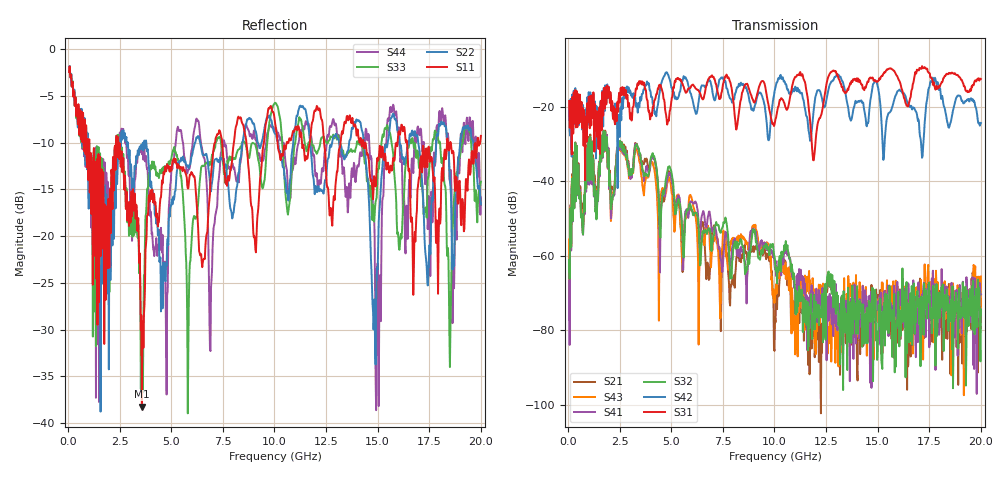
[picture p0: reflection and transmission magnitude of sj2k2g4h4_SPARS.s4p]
! FILE: E:\users\goganessyan\GBX_Backplane\FR408_backplane\1m_OUTBOUND_FEXT\sj2k2g4h4_SPARS.s4p
# MHZ S RI R 50.00
! FREQ  S11  S12  S13  S14
!  S21  S22  S23  S24
!  S31  S32  S33  S34
!  S41  S42  S43  S44
!  REAL  IMAG  REAL  IMAG  REAL  IMAG  REAL  IMAG
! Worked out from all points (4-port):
!   799 points, 50 MHz to 20 GHz, reference 50 ohm
!   strongest paths, dB at 50 MHz, 5.025 GHz, 10.03 GHz, 15.03 GHz, 20 GHz:
!     S31: -18.4, -17.5, -23.9, -13.1, -12.5
!     S42: -19.3, -15.0, -15.3, -15.0, -24.3
!     S32: -61.2, -38.0, -61.2, -81.1, -74.4
!     S41: -66.6, -40.3, -63.5, -72.2, -70.4
!     S43: -55.6, -43.4, -71.8, -78.0, -65.6
!     S21: -64.2, -40.0, -76.7, -70.5, -71.6
!   lowest |S11| = -38.2 dB at 3.575 GHz (marker M1), VSWR 1.02, Z = 49 + j0.704 ohm
!   |S11| at or under -10 dB: 2.433 GHz to 7.126 GHz (4.692 GHz wide, 98.2 % of centre); 14.31 GHz to 15.96 GHz (1.654 GHz wide, 10.9 % of centre); 16.42 GHz to 18.36 GHz (1.937 GHz wide, 11.1 % of centre)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
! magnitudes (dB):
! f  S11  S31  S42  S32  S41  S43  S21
! 50 MHz  -2.5  -18.4  -19.3  -61.2  -66.6  -55.6  -64.2
! 350 MHz  -5.1  -15.5  -14.9  -29.7  -30.3  -30.1  -29.5
! 3.575 GHz  -38.2  -14.0  -16.5  -35.1  -35.9  -39.1  -34.5
! 11.57 GHz  -11.7  -16.4  -22.6  -77.0  -85.3  -69.6  -76.1
! 14.97 GHz  -11.7  -13.2  -13.9  -88.0  -74.6  -74.1  -76.2
! 15.68 GHz  -13.0  -9.8  -20.6  -74.6  -74.7  -76.6  -82.4
! 20 GHz  -9.3  -12.5  -24.3  -74.4  -70.4  -65.6  -71.6
